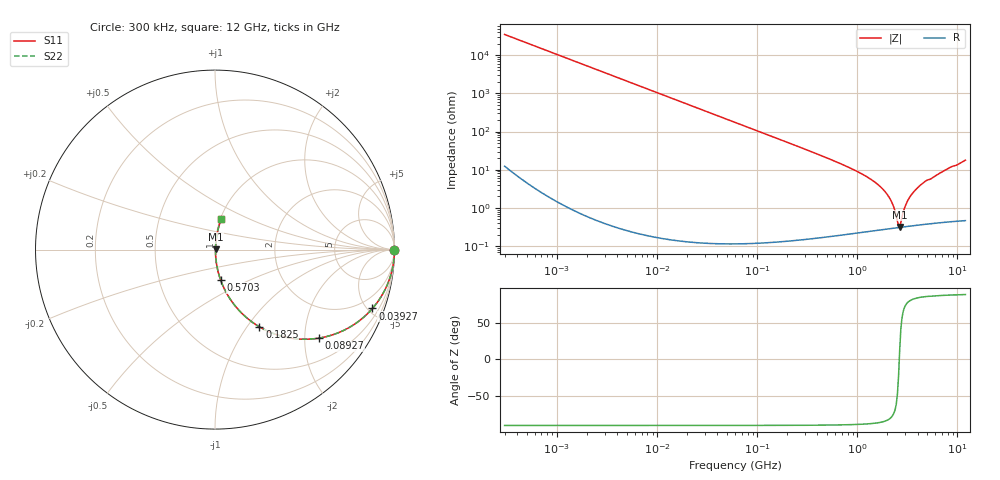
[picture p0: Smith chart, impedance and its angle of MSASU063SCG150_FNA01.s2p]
! MSASU063SCG150_FNA01  S-PARAMETER MODEL  ( Standard Model )
! Model Generated by TAIYO YUDEN Corporation (http://www.ty-top.com)
! Version 1.0
! TAIYO YUDEN Control No. 240819
! Copyright(c) 2024 TAIYO YUDEN CO.,LTD. All Rights Reserved.
! Product Description (link to TY-COMPAS)
! https://ds.yuden.co.jp/TYCOMPAS/or/detail?pn=MSASU063SCG150JFNA01&u=M
! Products Name : Multilayer Ceramic Capacitors
! Characteristics :
!  Capacitance : 15 [pF] , Rated Voltage : 50 [V] , TCC : CG / C0G
!  Case Size : 0.6 x 0.3 / 0.024 x 0.012 [mm/inch] , Thickness : 0.3 / 0.012 [mm/inch]
!  (Conditions: Temperature = 25 [degC] , DC Bias Voltage = 0 [V])
! External Node Assignments :
!  1  o---| |---o  2
! GND o---------o GND
! Frequency Range : 0.3MHz  -  12000MHz  [ 401 STEP ]
# MHZ S RI R 50
! Freq[MHz].  S11 Real  S11 Imag  S21 Real  S21 Imag  S12 Real  S12 Imag  S22 Real  S22 Imag
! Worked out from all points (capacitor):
!   401 points, 300 kHz to 12 GHz, reference 50 ohm
!   read as one part in series: C = 15.1 pF near 316.3 kHz
!   lowest |Z| = 318 mohm at 2.651 GHz (marker M1)
!   series resonance near 2.625 GHz, so ESL is about 240 pH
!   S11 on the Smith chart (normalised r, x): 300 kHz: open; 39.27 MHz: 1.00, -5.35; 89.27 MHz: 1.00, -2.35; 182.5 MHz: 1.00, -1.15; 570.3 MHz: 1.00, -0.35; 12 GHz: 1.01, +0.36
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0.3  1 -0.00285  9.16e-06 0.00285  9.16e-06 0.00285  1 -0.00285
1.769972  0.9997 -0.0168  0.000286 0.0168  0.000286 0.0168  0.9997 -0.0168
10.44266  0.9902 -0.0984  0.0098 0.0984  0.0098 0.0984  0.9902 -0.0984
39.27072  0.8773 -0.3279  0.1227 0.3279  0.1227 0.3279  0.8773 -0.3279
60  0.7538 -0.4305  0.2462 0.4305  0.2462 0.4305  0.7538 -0.4305
89.27472  0.5801 -0.493  0.4199 0.493  0.4199 0.493  0.5801 -0.493
182.544  0.2476 -0.4305  0.7524 0.4305  0.7524 0.4305  0.2476 -0.4305
353.9943  0.0795 -0.2678  0.9205 0.2678  0.9205 0.2678  0.0795 -0.2678
570.2811  0.0315 -0.1697  0.9685 0.1697  0.9685 0.1697  0.0315 -0.1697
1366.97  0.00554 -0.0555  0.9945 0.0555  0.9945 0.0555  0.00554 -0.0555
1735.023  0.0038 -0.0338  0.9962 0.0338  0.9962 0.0338  0.0038 -0.0338
2088.533  0.00317 -0.0182  0.9968 0.0182  0.9968 0.0182  0.00317 -0.0182
2261.293  0.00305 -0.0118  0.9969 0.0118  0.9969 0.0118  0.00305 -0.0118
2514.07  0.00303 -0.00326  0.997 0.00326  0.997 0.00326  0.00303 -0.00326
2650.866  0.00308 0.000758  0.9969 -0.000758  0.9969 -0.000758  0.00308 0.000758
2722.03  0.00311 0.00282  0.9969 -0.00282  0.9969 -0.00282  0.00311 0.00282
2947.191  0.00327 0.00897  0.9967 -0.00897  0.9967 -0.00897  0.00327 0.00897
3190.978  0.0035 0.0152  0.9965 -0.0152  0.9965 -0.0152  0.0035 0.0152
4050.141  0.00471 0.0343  0.9953 -0.0343  0.9953 -0.0343  0.00471 0.0343
4747.894  0.0061 0.0489  0.9939 -0.0489  0.9939 -0.0489  0.0061 0.0489
7648.807  0.0139 0.0978  0.9861 -0.0978  0.9861 -0.0978  0.0139 0.0978
12000  0.035 0.1711  0.965 -0.1711  0.965 -0.1711  0.035 0.1711
